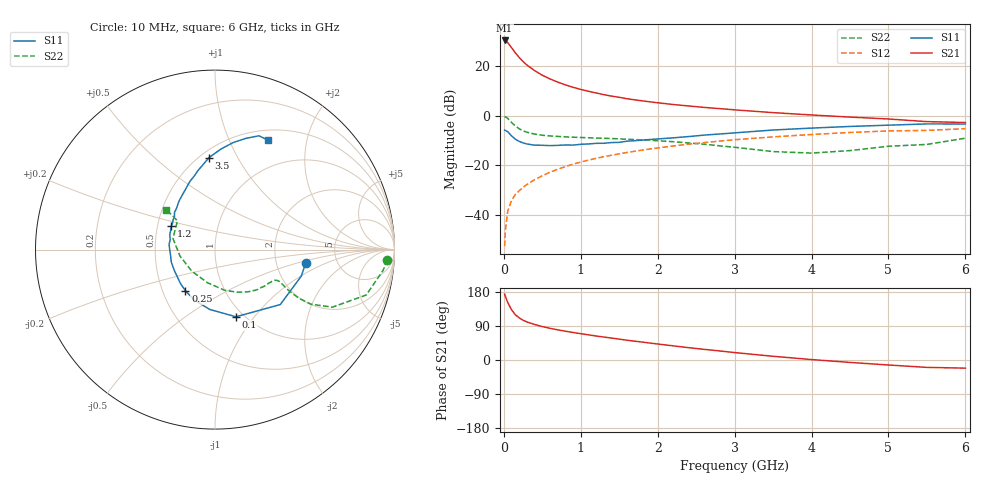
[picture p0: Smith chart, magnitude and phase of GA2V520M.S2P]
! Infineon Technologies  Discrete & RF Semiconductors
! BF775
! Si NPN RF Bipolar Junction Transistor in SOT23
! VCE = 2.5 V  IC = 20 mA
! Common Emitter S-Parameters:  May  1996
# GHz  S  MA  R  50
!  f  S11  S21  S12  S22
! GHz  MAG  ANG  MAG  ANG  MAG  ANG  MAG  ANG
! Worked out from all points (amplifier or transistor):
!   36 points, 10 MHz to 6 GHz, reference 50 ohm
!   highest |S21| = 30.1 dB at 10 MHz (marker M1)
!   |S21| within 3 dB of that: start of sweep to 103.1 MHz
!   unconditionally stable (mu >= 1): 357.9 MHz to 3.324 GHz
!   at 250 MHz: K = 0.89, MSG = 25.2 dB, |S12| = -28.8 dB
!   at 1.4 GHz: K = 1.13, MAG = 9.7 dB, |S12| = -15.9 dB
!   at 6 GHz: K = 0.98, MSG = 1.2 dB, |S12| = -5.3 dB
!   S11 on the Smith chart (normalised r, x): 10 MHz: 2.94, -0.61; 100 MHz: 0.92, -0.81; 250 MHz: 0.65, -0.33; 1.2 GHz: 0.59, +0.17; 3.5 GHz: 0.55, +0.77; 6 GHz: 0.62, +1.41
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0.01  0.5105 -8.6  32.11 173.9  0.0024 83.8  0.9617 -3.4
0.02  0.5031 -17.0  31.6 167.9  0.005 82.3  0.9434 -7.1
0.05  0.4755 -40.1  29.18 152.1  0.012 75.2  0.8798 -16.7
0.1  0.392 -72.7  23.09 132.5  0.0199 67.6  0.7287 -26.1
0.15  0.3347 -95.1  18.05 119.4  0.0261 65.1  0.6169 -29.6
0.2  0.3033 -112.5  14.62 111.1  0.0311 65.8  0.543 -30.1
0.25  0.2828 -125.6  12.11 104.9  0.0364 65.9  0.4943 -29.5
0.3  0.2691 -135.9  10.33 100.4  0.0414 67.5  0.4634 -28.9
0.4  0.255 -152.1  7.972 93.8  0.0517 68.5  0.4255 -27.3
0.5  0.2534 -164.1  6.432 88.2  0.0621 69.7  0.4026 -26.4
0.6  0.2495 -172.6  5.43 83.7  0.073 69.8  0.3901 -26.3
0.7  0.2524 -179.7  4.699 79.6  0.0838 70.0  0.3815 -26.6
0.8  0.2573 173.4  4.123 76.0  0.0945 69.0  0.3738 -27.2
0.9  0.2558 167.6  3.687 72.6  0.1062 68.8  0.368 -27.9
1.1  0.2693 156.8  3.072 66.4  0.1277 67.4  0.3589 -30.5
1.2  0.2774 151.5  2.837 63.3  0.1387 66.5  0.3537 -31.8
1.6  0.3065 137.4  2.176 52.2  0.1817 62.3  0.3349 -38.7
2.2  0.3574 120.1  1.667 37.4  0.2455 55.3  0.2992 -51.8
3.5  0.5131 93.8  1.145 9.8  0.3737 38.1  0.1894 -102.7
4.5  0.6048 80.4  0.932 -6.4  0.4581 24.3  0.1985 -169.7
5.5  0.6796 68.9  0.756 -19.5  0.504 9.5  0.2638 142.5
6  0.6781 64.0  0.726 -21.5  0.5461 5.2  0.3517 140.6
